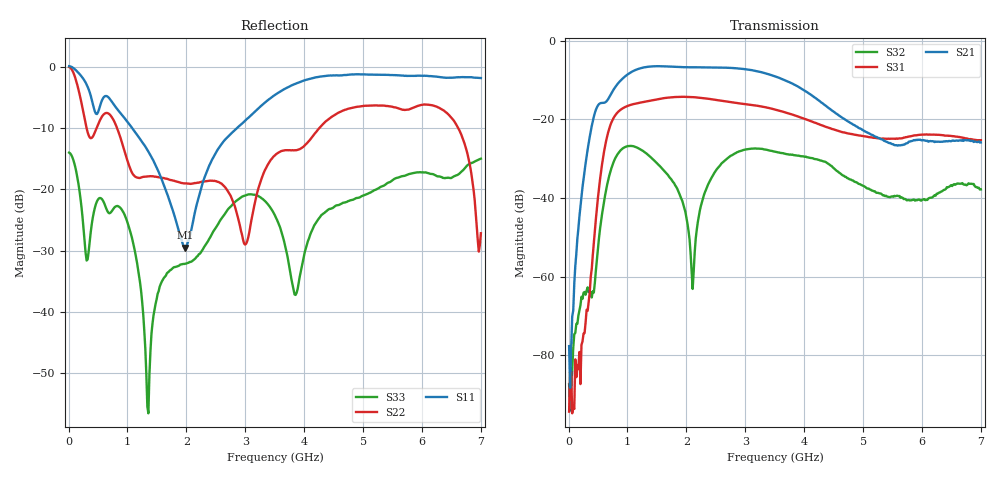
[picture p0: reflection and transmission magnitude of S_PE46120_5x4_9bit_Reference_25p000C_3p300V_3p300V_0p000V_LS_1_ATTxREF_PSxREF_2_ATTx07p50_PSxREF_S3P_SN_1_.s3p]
! Device ID: PE46120_5x4_9bit_Reference
! Device ID: PE46120_5x4_9bit_Reference
! File Path: z:\PE46120_5x4_9bit_Reference\MPAC_Yi\new_12port\25p000C\3p300\LS_1_ATTxREF_PSxREF_2_ATTx07p50_PSxREF\PE46120_5x4_9bit_Reference_25p000C_3p300V_3p300V_0p000V_LS_1_ATTxREF_PSxREF_2_ATTx07p50_PSxREF_S3P_SN_1_.s3p
! Serial: 1
! Lot:
! Temp: 25.000C
! VDD: 3.300
! VSS: 0.000
! Control_Hi: 3.300
! Control_Lo: 0.000
! Logic State: LS_1_ATTxREF_PSxREF_2_ATTx07p50_PSxREF
! Port 1: RFin
! Port 2: RFout1
! Port 3: RFout2
! ThroughPath:1-3
! IDD: -0.0005444512
! ISS: 0
! Comment:
#  Hz  S  RI  R  50
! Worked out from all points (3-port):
!   401 points, 10 MHz to 7 GHz, reference 50 ohm
!   strongest paths, dB at 10 MHz, 1.758 GHz, 3.505 GHz, 5.253 GHz, 7 GHz:
!     S21: -77.7, -6.6, -9.1, -24.7, -25.9
!     S31: -94.4, -14.4, -17.5, -24.8, -25.3
!     S32: -87.4, -35.6, -28.2, -38.7, -37.8
!   lowest |S11| = -29.5 dB at 1.985 GHz (marker M1), VSWR 1.07, Z = 53 + j1.74 ohm
!   |S11| at or under -10 dB: 1.077 GHz to 2.862 GHz (1.785 GHz wide, 90.6 % of centre)
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1e7  1 -0.1151  5.45e-05 3.53e-05  -0.000153 -1.39e-05
     4.12e-05 -0.000123  0.9863 -0.0969  -6.95e-05 7.9e-05
     1.82e-05 5.72e-06  -1.44e-05 4.02e-05  0.1981 -0.0167
2.5465e8  -0.5306 -0.5852  -0.0162 -0.00544  8.9e-05 0.000154
          -0.0165 -0.00554  -0.3208 -0.2657  -4.29e-05 0.000485
          7.41e-05 0.000173  -9.61e-05 0.000615  -0.0274 -0.0396
4.81825e8  -0.3999 -0.0902  -0.0431 0.1335  0.00717 0.00131
           -0.0434 0.135  0.1903 0.2571  -0.000903 0.00136
           0.00724 0.00126  -0.000806 0.00142  0.063 0.0486
9.5365e8  -0.2768 0.2581  0.3363 -0.0712  -0.0373 0.1356
          0.3398 -0.0725  -0.0521 -0.1951  -0.0204 0.0386
          -0.0376 0.1372  -0.0204 0.039  0.0435 -0.0438
1.3381e9  -0.087 0.1902  -0.0768 -0.4525  0.1675 -0.00278
          -0.078 -0.4573  -0.0645 -0.1098  0.0217 -0.0279
          0.1694 -0.00299  0.0219 -0.0285  -0.00164 -0.000429
1.984675e9  0.0292 0.0164  -0.3679 0.2663  -0.1161 -0.1511
            -0.3714 0.2694  -0.0903 0.0655  0.001 0.00657
            -0.118 -0.1526  0.00113 0.00648  0.0209 0.0134
2.107e9  0.0476 -0.0222  -0.257 0.3731  -0.1616 -0.0977
         -0.2595 0.3775  -0.0543 0.0973  0.000654 -0.000335
         -0.1638 -0.0985  0.000584 -0.000375  0.0205 0.0163
3.505e9  -0.4352 -0.3946  -0.0903 -0.3347  0.1297 0.0209
         -0.0917 -0.3389  0.0625 0.1786  0.0051 -0.0379
         0.1315 0.0207  0.00498 -0.0384  0.0611 0.000326
6.248575e9  -0.3748 0.7373  0.04 -0.0319  -0.00682 0.062
            0.0404 -0.0323  0.4618 -0.0944  -0.0117 -0.000607
            -0.00674 0.0632  -0.0112 -0.00086  0.1271 0.0171
7e9  -0.1108 0.7981  -0.0285 -0.0403  0.0478 0.0229
     -0.0295 -0.0413  -0.0377 0.0222  0.0104 0.0068
     0.049 0.0231  0.0107 0.00704  0.1222 0.1288
